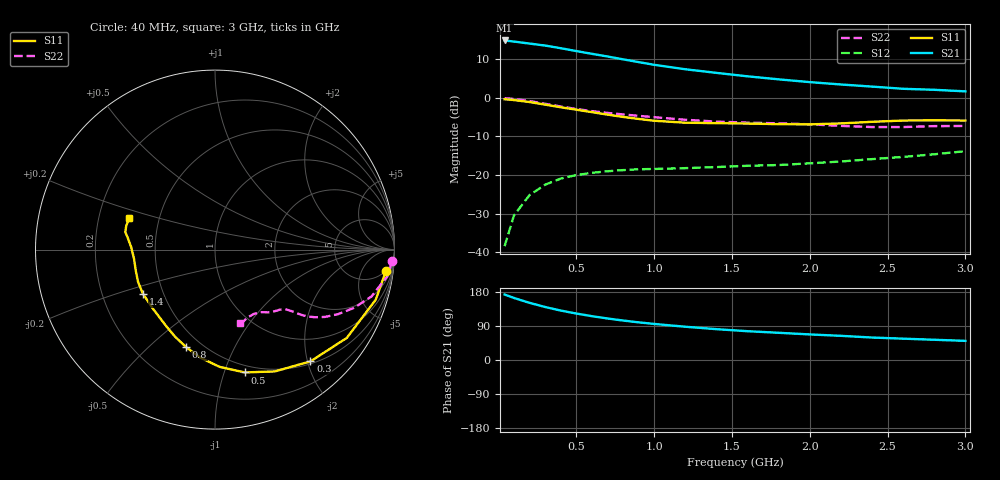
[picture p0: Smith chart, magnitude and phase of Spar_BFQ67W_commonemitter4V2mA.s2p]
! Filename:  BFQ67WA.S2P  Version:  4.0
! NXP part #: BFQ67W  Date: Jun 1994
! Bias condition: Vce=4V, Ic=2mA
#  MHz  S  MA  R  50
! Freq  S11  S21  S12  S22  !GUM [dB]
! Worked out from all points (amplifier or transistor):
!   21 points, 40 MHz to 3 GHz, reference 50 ohm
!   highest |S21| = 14.9 dB at 40 MHz (marker M1)
!   |S21| within 3 dB of that: start of sweep to 536 MHz
!   unconditionally stable (mu >= 1): 1.276 GHz to end of sweep
!   at 300 MHz: K = 0.29, MSG = 18.0 dB, |S12| = -22.5 dB
!   at 1 GHz: K = 0.81, MSG = 13.5 dB, |S12| = -18.4 dB
!   at 3 GHz: K = 1.15, MAG = 5.4 dB, |S12| = -13.8 dB
!   lowest NFmin = 1.30 dB at 1 GHz
!   S11 on the Smith chart (normalised r, x): 40 MHz: 5, -15; 300 MHz: 0.54, -2.05; 500 MHz: 0.43, -1.18; 800 MHz: 0.41, -0.66; 1.4 GHz: 0.38, -0.24; 3 GHz: 0.33, +0.16
40  0.96 -7.1  5.547 172.8  0.012 84.9  0.99 -3.7
100  0.938 -17.3  5.366 163.7  0.03 77.8  0.971 -8.9
200  0.884 -33.8  5.056 150.9  0.055 67.5  0.91 -16.7
300  0.819 -49.5  4.766 139.9  0.075 59.5  0.839 -22.8
400  0.756 -63.9  4.403 130.5  0.09 53.5  0.774 -27.7
500  0.704 -76.4  4.045 122.7  0.1 49.0  0.718 -31.5
600  0.654 -87.7  3.726 115.7  0.107 46.1  0.674 -34.0
700  0.608 -97.7  3.441 109.6  0.112 44.5  0.639 -35.7
800  0.567 -106.4  3.161 104.2  0.116 43.3  0.611 -36.8
900  0.534 -114.6  2.91 99.4  0.119 42.7  0.586 -37.6
1000  0.506 -122.4  2.685 95.2  0.12 42.7  0.563 -38.2
1200  0.477 -137.0  2.351 87.8  0.123 43.4  0.521 -39.9
1400  0.471 -148.5  2.111 81.4  0.127 45.4  0.493 -42.7
1600  0.465 -157.2  1.904 76.0  0.132 48.1  0.478 -45.9
1800  0.457 -164.9  1.739 71.8  0.135 52.0  0.468 -48.2
2000  0.454 -173.5  1.601 67.5  0.142 55.8  0.455 -50.2
2200  0.467 178.4  1.492 63.8  0.15 59.9  0.434 -53.4
2400  0.49 172.4  1.401 59.3  0.161 63.1  0.419 -58.6
2600  0.509 169.0  1.312 56.3  0.172 65.7  0.419 -64.5
2800  0.512 165.1  1.273 53.4  0.186 68.9  0.431 -68.6
3000  0.509 159.9  1.215 50.5  0.204 71.1  0.433 -71.2
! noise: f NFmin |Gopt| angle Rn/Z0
1000  1.3  0.75  73  0.215
